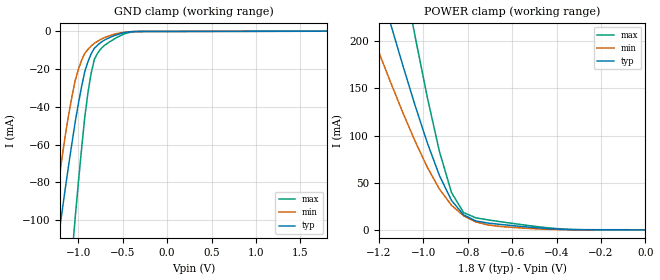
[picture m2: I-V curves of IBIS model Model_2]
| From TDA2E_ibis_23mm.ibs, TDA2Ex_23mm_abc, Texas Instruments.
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| Model based on original model for BMLBLVDS18_SSCEH
|   Sub model LVDS_RX_MODE_10P_1P8
[model]   Model_2
|[Description]  [1.8V-INPUT-LVDS MODE-X, IND, 10%]
|   LVDS MODE,IND,10%
|[Input Load]   LVDS MODE
|[Output Drive]
|Voltage   1.8V
|Mode   INPUT
Model_type   Input
Polarity   Non-Inverting
C_comp   3.4p   3.05p   3.82p
Vinl =  1.15V
Vinh =  1.25V
[Temperature Range]   25   125   -40
[Voltage Range]   1.8   1.62   1.98
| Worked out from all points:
|   GND clamp passes 1 mA (typ) near -0.51 V on its own axis
|   POWER clamp passes 1 mA (typ) near -0.40 V on its own axis
[POWER_clamp]
-1.8V     779.9mA    580mA      1.224A
-1.236V   292.1mA    211mA      460.4mA
-1.145V   217.2mA    155.6mA    341.7mA
-1.127V   202.7mA    145mA      318.5mA
-1.055V   145.7mA    103.9mA    227.2mA
-1.036V   131.7mA    93.91mA    204.8mA
-927.3mV  57.78mA    43.43mA    83.32mA
-872.7mV  31.31mA    26.15mA    39.61mA
-818.2mV  16.05mA    15.08mA    18.46mA
-709.1mV  7.358mA    5.366mA    10.74mA
-600mV    4.702mA    2.795mA    7.071mA
0V        145uA      51.95uA    279uA
[GND_clamp]
-1.8V     -321.4mA   -309.3mA   -563.9mA
-1.291V   -133.4mA   -105mA     -247.9mA
-1.218V   -107.9mA   -79mA      -204.2mA
-1.073V   -59.81mA   -35.07mA   -120mA
-1.036V   -48.68mA   -26.51mA   -99.89mA
-927.3mV  -21.51mA   -11.71mA   -45.86mA
-890.9mV  -16.08mA   -9.545mA   -32.61mA
-818.2mV  -8.944mA   -6.331mA   -14.73mA
-781.8mV  -7.267mA   -5.249mA   -11.59mA
-600mV    -2.366mA   -1.608mA   -4.187mA
-381.8mV  -124.6uA   -112.9uA   -234.8uA
1.8V      145uA      118uA      146.8uA
